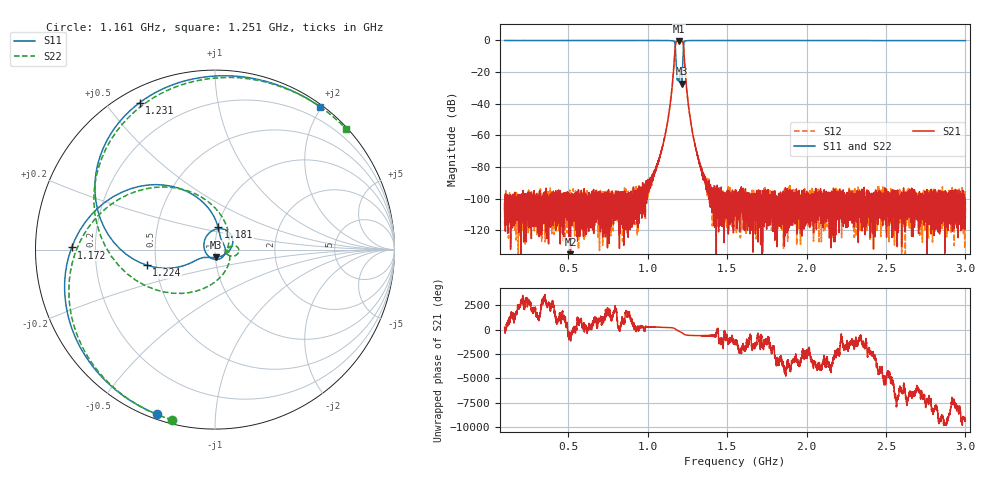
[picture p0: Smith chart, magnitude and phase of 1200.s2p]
# Hz S DB R 50
! Planar, S50180, 20087770, 20.1.2/1
! Date: 23.06.2021 14:42:00
! Data: Format (Calibration Info)
! Freq	S11:dB/Ang(F2)	S21:dB/Ang(F2)	S12:dB/Ang(F2)	S22:dB/Ang(F2)
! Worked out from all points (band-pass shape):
!   8991 points, 100 MHz to 3 GHz, reference 50 ohm
!   highest |S21| = -0.42 dB at 1.196 GHz (marker M1); lowest = -154.8 dB at 514.5 MHz (marker M2)
!   |S21| within 3 dB of the highest: 1.174 GHz to 1.226 GHz (51.58 MHz wide, 4.3 % of centre)
!   lowest |S11| = -27.2 dB at 1.215 GHz (marker M3), VSWR 1.09, Z = 50.6 - j4.34 ohm
!   |S11| at or under -10 dB: 1.178 GHz to 1.223 GHz (45.11 MHz wide, 3.76 % of centre)
!   |S22| runs from -24.4 to 0.0 dB; largest |S21 - S12| = 0.018
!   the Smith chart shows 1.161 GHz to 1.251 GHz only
!   S11 on the Smith chart (normalised r, x): 1.161 GHz: 0.02, -0.71; 1.172 GHz: 0.11, +0.01; 1.181 GHz: 1.00, +0.25; 1.224 GHz: 0.44, -0.09; 1.231 GHz: 0.06, +0.61; 1.251 GHz: 0.03, +1.98
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1e8  0.02 154.0  -108.27 154.3  -103.16 173.4  0.01 150.3
2.945161e8  -0.03 108.0  -98.80 25.9  -107.58 74.1  -0.00 99.6
5.145161e8  -0.01 65.2  -154.78 0.7  -102.70 110.5  -0.01 56.5
5.835484e8  -0.01 54.3  -115.69 -175.1  -112.48 132.0  0.01 45.2
1.066774e9  -0.01 -24.2  -76.48 -121.8  -75.85 -120.0  0.03 -27.7
1.123871e9  -0.03 -50.7  -52.49 -142.2  -52.57 -142.7  -0.02 -51.2
1.149677e9  -0.11 -81.2  -33.84 -171.9  -33.84 -172.1  -0.07 -78.3
1.160645e9  -0.24 -109.4  -22.21 160.4  -22.21 160.3  -0.19 -104.0
1.171935e9  -1.95 179.1  -6.30 88.0  -6.30 87.9  -1.94 -174.5
1.180968e9  -18.05 82.0  -0.62 -26.5  -0.63 -26.7  -18.58 50.3
1.196129e9  -25.60 -146.7  -0.42 -162.3  -0.42 -162.4  -23.22 -1.1
1.205806e9  -18.08 59.3  -0.48 119.8  -0.48 119.7  -17.51 -2.6
1.214516e9  -27.24 -80.2  -0.47 44.5  -0.48 44.5  -24.42 -8.7
1.223548e9  -8.16 -167.2  -1.52 -58.5  -1.52 -58.5  -8.65 -140.3
1.23129e9  -0.72 117.1  -11.57 -151.7  -11.58 -151.7  -0.79 111.9
1.25129e9  -0.11 53.6  -36.16 140.1  -36.15 140.1  -0.06 42.6
1.288065e9  -0.02 20.3  -61.02 105.9  -61.02 106.0  -0.00 10.6
1.336129e9  -0.01 2.5  -79.72 87.7  -80.75 89.6  -0.00 -6.1
1.55e9  -0.01 -30.2  -104.24 -45.1  -104.74 -126.2  0.03 -35.6
2.033548e9  -0.04 -72.1  -102.71 -137.6  -93.50 60.6  -0.01 -73.8
2.516774e9  -0.07 -108.0  -108.06 -80.5  -107.82 134.9  -0.05 -106.7
3e9  -0.11 -144.3  -103.27 60.4  -104.17 156.1  -0.09 -140.3
